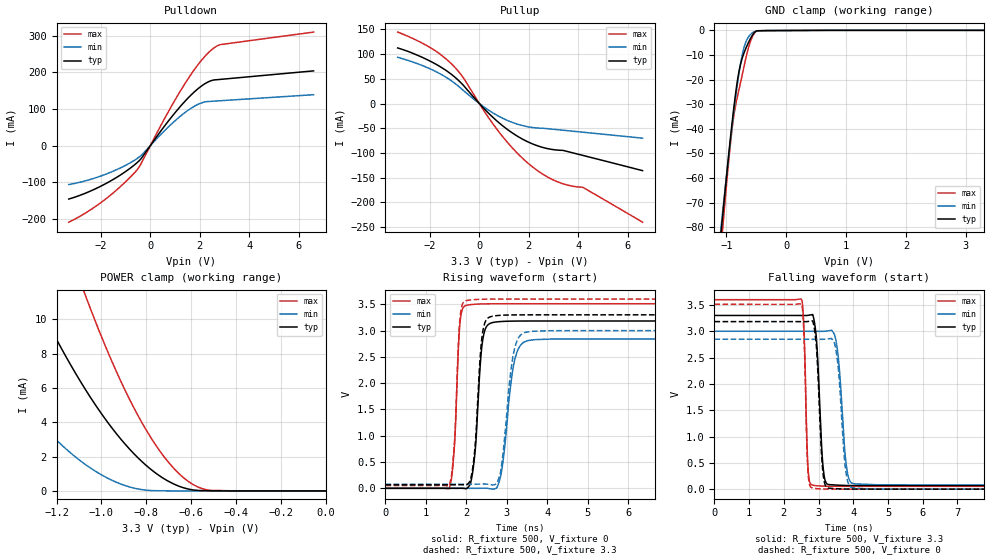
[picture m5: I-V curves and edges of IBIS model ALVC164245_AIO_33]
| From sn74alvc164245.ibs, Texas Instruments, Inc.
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[Model]   ALVC164245_AIO_33
Model_type  I/O
Vinl=0.8
Vinh=2
Enable   Active-Low
Vref =   0
Rref =   500
Cref =   30p
Vmeas =   1.65
| variable   typ   min   max
C_comp   8.5pF   NA   NA
| C_pullup   3.20pF   2.71pF   3.75pF
| C_pulldown   3.31pF   2.64pF   4.26pF
| C_tri-state   2.91pF   2.49pF   3.57pF
[Temperature Range]   40   100   -40
| Ambient temperature   25   85   -40
[Voltage range]   3.3   3   3.6
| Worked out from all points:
|   slope of the pulldown table from 0 to 0.495 V, typ, clamps not added: 10.7 ohm
|   slope of the pullup table from 0 to 0.495 V, typ, clamps not added: 19.5 ohm
|   GND clamp passes 1 mA (typ) near -0.54 V on its own axis
|   POWER clamp passes 1 mA (typ) near -0.75 V on its own axis
|   rising waveform, R_fixture 500, V_fixture 0: 20-80 % time 156ps typ, 237ps min, 117ps max; typ from 0 V to 3.18 V
|   falling waveform, R_fixture 500, V_fixture 3.3: 20-80 % time 138ps typ, 184ps min, 84.8ps max; typ from 3.3 V to 0.067 V
|   rising waveform, R_fixture 500, V_fixture 3.3: 20-80 % time 152ps typ, 226ps min, 118ps max; typ from 0.067 V to 3.3 V
|   falling waveform, R_fixture 500, V_fixture 0: 20-80 % time 134ps typ, 175ps min, 83.2ps max; typ from 3.18 V to 0 V
[GND Clamp]
| ALVC164245_AIO_33
|   Voltage   I(typ)   I(min)   I(max)
-3.3V     -724.5mA   -661.5mA   -819.8mA
-1.105V   -86.29mA   -83.67mA   -93.18mA
-1.08V    -79.83mA   -77.81mA   -85.86mA
-1.06V    -74.72mA   -73.17mA   -80.07mA
-915mV    -39.73mA   -41.03mA   -42.12mA
-865mV    -29.19mA   -30.91mA   -33.08mA
-805mV    -18.81mA   -19.95mA   -25.69mA
-750mV    -12.49mA   -11.73mA   -19.65mA
-690mV    -8.181mA   -5.715mA   -12.93mA
-545mV    -1.258mA   -688uA     -1.566mA
-420mV    -110.6uA   -127.7uA   -157uA
3.3V      15.97uA    12.63uA    25.22uA
[POWER Clamp]
| ALVC164245_AIO_33
|   Voltage   I(typ)   I(min)   I(max)
-3.3V     94.55mA    63.57mA    143.1mA
-1.69V    23.53mA    11.7mA     38.87mA
-1.66V    22.5mA     11.03mA    37.33mA
-1.47V    16.32mA    7.187mA    28.01mA
-1.295V   11.28mA    4.267mA    20.14mA
-1.07V    5.89mA     1.528mA    11.36mA
-950mV    3.619mA    602.3uA    7.457mA
-840mV    1.969mA    122.8uA    4.471mA
-735mV    828.7uA    9.289uA    2.242mA
-635mV    187.2uA    1.143uA    781.2uA
-510mV    6.192uA    101nA      32.11uA
-48.03fV  1.723nA    15.12nA    4.768nA
[Pulldown]
| ALVC164245_AIO_33
|   Voltage   I(typ)   I(min)   I(max)
-3.3V     -146.2mA   -106.5mA   -209.5mA
-2.625V   -130.2mA   -96.47mA   -184.4mA
-1.88V    -106.7mA   -80.21mA   -149.9mA
-1.205V   -80.18mA   -60.89mA   -111.8mA
-570mV    -48.66mA   -37.01mA   -69.12mA
-400mV    -37.66mA   -28.54mA   -52.46mA
740mV     68.11mA    51.7mA     94.11mA
1.395V    120.8mA    90.04mA    169mA
2.01V     160mA      115.1mA    228.4mA
2.525V    178.7mA    121.2mA    264.6mA
2.875V    181.2mA    122.8mA    276.6mA
6.6V      204.2mA    139.1mA    310.3mA
[Pullup]
| ALVC164245_AIO_33
|   Voltage   I(typ)   I(min)   I(max)
-3.3V     112.4mA    93.41mA    144.4mA
-1.965V   85.08mA    69.55mA    112.5mA
-1.085V   57.25mA    44.34mA    78.09mA
-635mV    36.2mA     26mA       51.16mA
155mV     -8.395mA   -5.804mA   -12.16mA
675mV     -33.67mA   -22.63mA   -49.58mA
1.425V    -62.43mA   -39.82mA   -94.6mA
2.175V    -82.1mA    -48.64mA   -129mA
2.675V    -90.15mA   -50.46mA   -146.1mA
3.175V    -94.17mA   -52.93mA   -158.5mA
4.175V    -104.7mA   -57.89mA   -169.1mA
6.6V      -135.6mA   -70mA      -239.8mA
[Ramp]
| ALVC164245_AIO_33
| variable   typ   min   max
dV/dt_r   1.92/1.59E-10   1.71/2.46E-10   2.11/1.19E-10
dV/dt_f   1.95/1.48E-10   1.76/1.94E-10   2.13/8.86E-11
R_load = 500
[Rising Waveform]
| ALVC164245_AIO_33
R_fixture =   500
C_fixture =   0
L_fixture =   0
V_fixture =   0
V_fixture_min = 0
V_fixture_max = 0
|   Time   V(typ)   V(min)   V(max)
0s        201.9pV    3.297nV    119.3nV
1.57ns    -45.64uV   9.689uV    -8.596mV
1.705ns   -22.13uV   -8.133uV   801.8mV
1.855ns   957.9uV    -20.41uV   3.234V
2.15ns    278mV      -59.62uV   3.498V
2.41ns    2.848V     1.489mV    3.508V
2.81ns    3.17V      120mV      3.511V
3.21ns    3.181V     2.488V     3.511V
3.71ns    3.183V     2.829V     3.511V
50ns      3.183V     2.842V     3.511V
[Falling Waveform]
| ALVC164245_AIO_33
R_fixture =   500
C_fixture =   0
L_fixture =   0
V_fixture =   3.3
V_fixture_min = 3
V_fixture_max = 3.6
|   Time   V(typ)   V(min)   V(max)
0s        3.3V       3V         3.6V
2.51ns    3.299V     3V         3.604V
2.58ns    3.299V     3V         3.022V
2.705ns   3.303V     3V         327.2mV
2.93ns    2.924V     2.999V     66.57mV
3.18ns    186.2mV    3V         57.23mV
3.495ns   78.29mV    2.845V     54.71mV
3.8ns     70.41mV    452.7mV    54.05mV
4.02ns    68.58mV    101.9mV    53.88mV
50ns      67.07mV    79mV       53.65mV
[Rising Waveform]
| ALVC164245_AIO_33
R_fixture =   500
C_fixture =   0
L_fixture =   0
V_fixture =   3.3
V_fixture_min = 3
V_fixture_max = 3.6
|   Time   V(typ)   V(min)   V(max)
0s        67.06mV    78.99mV    53.64mV
1.57ns    67.02mV    79mV       45.42mV
1.71ns    67.06mV    78.98mV    925.8mV
1.855ns   67.93mV    78.97mV    3.325V
2.115ns   203.9mV    78.95mV    3.584V
2.405ns   2.978V     80.31mV    3.597V
2.775ns   3.287V     130.1mV    3.6V
3.185ns   3.299V     2.634V     3.6V
3.63ns    3.3V       2.986V     3.6V
50ns      3.3V       3V         3.6V
[Falling Waveform]
| ALVC164245_AIO_33
R_fixture =   500
C_fixture =   0
L_fixture =   0
V_fixture =   0
V_fixture_min = 0
V_fixture_max = 0
|   Time   V(typ)   V(min)   V(max)
0s        3.183V     2.848V     3.511V
2.51ns    3.182V     2.848V     3.512V
2.7ns     3.186V     2.848V     284.8mV
2.92ns    2.841V     2.847V     12.3mV
3.11ns    429mV      2.847V     4.64mV
3.285ns   19.69mV    2.856V     1.963mV
3.53ns    8.576mV    2.515V     832.5uV
3.81ns    2.608mV    237.3mV    348.4uV
4.055ns   1.108mV    20.77mV    194.9uV
50ns      6.561uV    10.46uV    7.653uV
